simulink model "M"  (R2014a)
settings: Solver=FixedStepDiscrete  StartTime=0.0  StopTime=1  FixedStep=0.02/40  RelTol=1e-3
undefined symbols (not defined in the file or in its folder): D11, Delta
libraries: powerlib x10

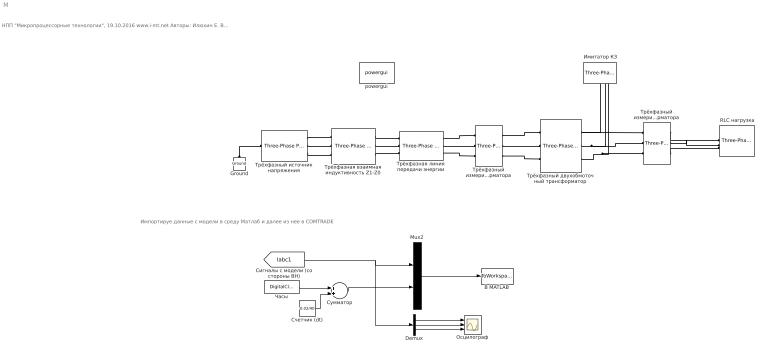
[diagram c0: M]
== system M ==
  note: Импортируе данные с модели в среду Матлаб и далее из нее в COMTRADE
  note: НПП "Микропроцессорные технологии", 19.10.2016 www.i-mt.net Авторы: Илюхин Е. В., Пирогов М. Г. Если вы скачали этот файл, мы рады и желаем вам творческого развития на благо инженерной мысли и научно-технического прогресса! P.S. для пониманя всех тонкостей и нюансов изучите выбранные нами настройки режима моделирования системы
  " RLC нагрузка" : powerlib/Elements/Three-Phase Parallel RLC Load  LConnTagsString=A|B|C  Configuration=Delta  NominalVoltage=6000  NominalFrequency=50  ActivePower=2.5e6  InductivePower=100  CapacitivePower=100  Measurements=None  LoadType=constant Z
  " Имитатор КЗ" : powerlib/Elements/Three-Phase Fault  InitialStates=0  FaultA=on  FaultB=off  FaultC=on  GroundFault=off  SwitchTimes=[0.3 0.4 0.6]  External=off  SwitchStatus=NaN  FaultResistance=0.002  GroundResistance=0.2  SnubberResistance=1e6  SnubberCapacitance=inf  Measurements=None
  Demux : Demux  Outputs=3
  Ground : powerlib/Elements/Ground  LConnTagsString=a
  Mux2 : Mux  Inputs=2
  powergui : powerlib/powergui  Priority=1  SimulationMode=Discrete  SolverType=Tustin  SampleTime=0.02/40  frequency=60  SPID=off  DisableSnubberDevices=off  DisableRonSwitches=off  DisableVfSwitches=off  SwTol=0  Interpol=off  DisplayEquations=off  Ts=0  methode=off  frequencyindice=0  Pbase=100e6  ErrMax=1e-4  Iterations=50  UnitsV=kV  UnitsW=MW  FunctionMessages=off  echomessages=off  HookPort=off  EnableUseOfTLC=off  x0status=blocks  RestoreLinks=warning  ResistiveCurrentMeasurement=off  Frange=[0:2:500]  Ylog=off  Xlog=on  ShowGrid=off  save=off  variable=ZData  structure=0  ZoomFFT=on  StartTime=0.0  cycles=1  DisplayStyle=1  fundamental=60  FreqAxis=off  MaxFrequency=1000  frequencyindicesteady=1  RmsSteady=1  display=off
  В MATLAB : ToWorkspace  VariableName=DATA  SampleTime=-1
  Осцилограф : Scope  NumInputPorts=3
  Сумматор : Sum
  Счетчик (dt) : Constant  Value=0.02/40
  Трёхфазная взаимная индуктивность Z1-Z0 : powerlib/Elements/Three-Phase Mutual Inductance Z1-Z0  LConnTagsString=a|b|c  RConnTagsString=A|B|C  PositiveSequence="[0.33  41e-3]"  ZeroSequence="[0.35  95e-3]"
  Трёхфазная линия передачи энергии : powerlib/Elements/Three-Phase PI Section Line  LConnTagsString=a|b|c  RConnTagsString=A|B|C  Frequency=60  Resistances=[ 0.01273 0.3864]  Inductances="[ 0.9337e-3  4.1264e-3]"  Capacitances=[12.74e-9 7.751e-9]  Length=100
  Трёхфазный двухобмоточный трансформатор : powerlib/Elements/Three-Phase Transformer (Two Windings)  Winding1Connection=Yg  UNITS=pu  NominalPower=[6.3e6 , 50 ]  Winding1=[ 115e3 , 0.002 , 0.08 ]  Winding2Connection=Delta (D11)  Winding2=[ 6.6e3 , 0.002 , 0.08 ]  SetSaturation=off  Rm=500  Lm=500  Saturation=[ 0,0 ; 0.0024,1.2 ; 1.0,1.52 ]  Hysteresis=off  DataFile='hysteresis'  SetInitialFlux=off  InitialFluxes=[ 0.8 , -0.8 , 0.7 ]  Measurements=None  MoreParameters=off  BreakLoop=off  DataType=off  TransfoNumber=1
  Трёхфазный измеритель тока и напряжения на стороне ВН трансформатора : powerlib/Measurements/Three-Phase V-I Measurement  VoltageMeasurement=phase-to-ground  SetLabelV=on  LabelV=Vabc1  Vpu=off  VpuLL=off  CurrentMeasurement=yes  SetLabelI=on  LabelI=Iabc1  Ipu=off  Pbase=100e6  Vbase=500e3  OutputType=Complex  PhasorSimulation=off  PSBequivalent=0
  Трёхфазный измеритель тока и напряжения на стороне НН трансформатора : powerlib/Measurements/Three-Phase V-I Measurement  VoltageMeasurement=phase-to-phase  SetLabelV=on  LabelV=Vabc2  Vpu=off  VpuLL=off  CurrentMeasurement=yes  SetLabelI=on  LabelI=Iabc2  Ipu=off  Pbase=100e6  Vbase=500e3  OutputType=Complex  PhasorSimulation=off  PSBequivalent=0
  Трёхфазный источник напряжения : powerlib/Electrical Sources/Three-Phase Programmable Voltage Source  PositiveSequence="[110e3  0 50]"  VariationEntity=None  VariationType=Step  VariationTypeAlt=Ramp  VariationStep=-25  VariationRate=-0.2  VariationMagnitude=0.3  VariationFrequency=2  VariationTiming=[0.1 11]  VariationPhaseA=off  Amplitudes=[1 0.8 1.2 1.0]  TimeValues=[0 0.1 0.15 0.2]  HarmonicGeneration=off  HarmonicA=[3 0.2 -25 0]  HarmonicB=[2 0.15 35 2]  Timing="[0.05  3]"  BusType=swing  Pref=0  Qref=0  Qmin=-inf  Qmax=inf
  Часы : DigitalClock  SampleTime=0.02/40
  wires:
  Mux2/1 -> В MATLAB/1
  [Iabc1] -> Demux/1, Mux2/1
  Часы/1 -> Сумматор/1
  Счетчик (dt)/1 -> Сумматор/2
  Сумматор/1 -> Mux2/2
  Demux/1 -> Осцилограф/1
  Demux/2 -> Осцилограф/2
  Demux/3 -> Осцилограф/3
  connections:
  Трёхфазный источник напряжения/RConn3 -- Трёхфазная взаимная индуктивность Z1-Z0/LConn3
  Трёхфазная взаимная индуктивность Z1-Z0/LConn2 -- Трёхфазный источник напряжения/RConn2
  Трёхфазный источник напряжения/RConn1 -- Трёхфазная взаимная индуктивность Z1-Z0/LConn1
  Ground/LConn1 -- Трёхфазный источник напряжения/LConn1
  Трёхфазный измеритель тока и напряжения на стороне НН трансформатора/LConn1 -- " RLC нагрузка"/LConn1
  Трёхфазный измеритель тока и напряжения на стороне НН трансформатора/LConn2 -- " RLC нагрузка"/LConn2
  Трёхфазный измеритель тока и напряжения на стороне НН трансформатора/LConn3 -- " RLC нагрузка"/LConn3
  Трёхфазный измеритель тока и напряжения на стороне ВН трансформатора/RConn1 -- Трёхфазный двухобмоточный трансформатор/LConn1
  Трёхфазный измеритель тока и напряжения на стороне ВН трансформатора/RConn2 -- Трёхфазный двухобмоточный трансформатор/LConn2
  Трёхфазный измеритель тока и напряжения на стороне ВН трансформатора/RConn3 -- Трёхфазный двухобмоточный трансформатор/LConn3
  Трёхфазный двухобмоточный трансформатор/RConn1 -- " Имитатор КЗ"/LConn1 -- Трёхфазный измеритель тока и напряжения на стороне НН трансформатора/RConn1
  Трёхфазный двухобмоточный трансформатор/RConn2 -- " Имитатор КЗ"/LConn2 -- Трёхфазный измеритель тока и напряжения на стороне НН трансформатора/RConn2
  Трёхфазный двухобмоточный трансформатор/RConn3 -- " Имитатор КЗ"/LConn3 -- Трёхфазный измеритель тока и напряжения на стороне НН трансформатора/RConn3
  Трёхфазная линия передачи энергии/RConn1 -- Трёхфазный измеритель тока и напряжения на стороне ВН трансформатора/LConn1
  Трёхфазная линия передачи энергии/RConn2 -- Трёхфазный измеритель тока и напряжения на стороне ВН трансформатора/LConn2
  Трёхфазная линия передачи энергии/RConn3 -- Трёхфазный измеритель тока и напряжения на стороне ВН трансформатора/LConn3
  Трёхфазная взаимная индуктивность Z1-Z0/RConn1 -- Трёхфазная линия передачи энергии/LConn1
  Трёхфазная взаимная индуктивность Z1-Z0/RConn2 -- Трёхфазная линия передачи энергии/LConn2
  Трёхфазная взаимная индуктивность Z1-Z0/RConn3 -- Трёхфазная линия передачи энергии/LConn3
